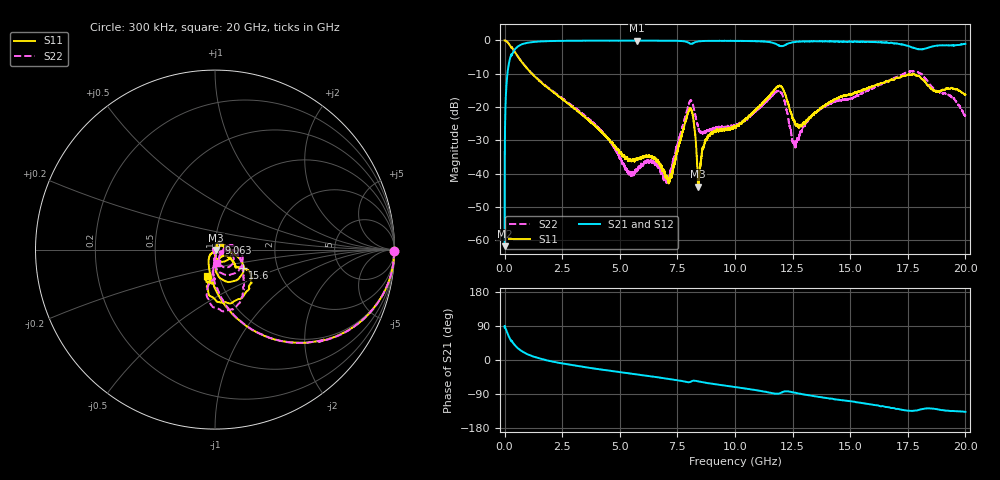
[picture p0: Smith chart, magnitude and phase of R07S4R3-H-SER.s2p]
!{R07S4R3}
!Johanson Technology Inc.
!www.johansontechnology.com
!Test Board Conditions:
!Substrate Type  RO4350B
!Substrate Thickness  10 mil
!Substrate Dk  3.66
!TL Type: GCPW
!TL Trace Width  21 mil
!TL Gap  20 mil
!Electrode orientation  Horizontal
!DUT TOPOLOGY	SERIES
!Mounting Pad LxW  16x21 mil
! Created Sat Feb  6 11:33:24 2021
# hz S ma R 50
! 2 Port Network Data from SP1.SP block
! freq  magS11  angS11  magS21  angS21  magS12  angS12  magS22  angS22
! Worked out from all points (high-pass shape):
!   20001 points, 300 kHz to 20 GHz, reference 50 ohm
!   highest |S21| = -0.04 dB at 5.74 GHz (marker M1); lowest = -61.7 dB at 300 kHz (marker M2)
!   |S21| within 3 dB of the highest: 408.8 MHz to end of sweep
!   lowest |S11| = -43.8 dB at 8.403 GHz (marker M3), VSWR 1.01, Z = 50.6 - j0.231 ohm
!   |S11| at or under -10 dB: 1.19 GHz to end of sweep
!   |S22| runs from -42.8 to 0.0 dB; largest |S21 - S12| = 0.013
!   S11 on the Smith chart (normalised r, x): 300 kHz: open; 9.063 GHz: 1.04, +0.08; 15.6 GHz: 1.33, -0.28; 20 GHz: 0.88, -0.26
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300000  0.9998 -0.5  0.0008196 86.0  0.00085 84.6  1 -0.6
1.163e8  0.9523 -18.5  0.3014 71.8  0.3017 71.7  0.9524 -18.4
3.463e8  0.7574 -42.6  0.6424 46.9  0.6437 47.0  0.7574 -42.5
1.1543e9  0.3255 -78.9  0.9402 11.2  0.9403 11.1  0.3293 -77.8
3.3343e9  0.0784 -116.8  0.9916 -17.4  0.9917 -17.4  0.08231 -94.5
5.4083e9  0.01628 -103.7  0.9934 -35.4  0.9939 -35.4  0.01018 -147.0
5.7403e9  0.0164 -81.2  0.9953 -38.1  0.9939 -38.1  0.01115 171.0
6.6673e9  0.01551 -64.4  0.9928 -45.8  0.9926 -45.9  0.01226 132.8
7.1843e9  0.008988 2.2  0.9909 -50.3  0.9897 -50.3  0.01005 39.3
8.0543e9  0.0953 -22.9  0.8957 -58.0  0.8962 -58.0  0.1249 -35.2
8.2063e9  0.06073 -72.9  0.918 -54.5  0.9178 -54.6  0.09903 -68.1
8.4033e9  0.006436 -20.8  0.9673 -56.3  0.9661 -56.4  0.04869 -62.9
8.6733e9  0.02803 65.2  0.9819 -59.5  0.9817 -59.5  0.04272 -39.2
9.0633e9  0.04231 60.8  0.9864 -63.3  0.9858 -63.3  0.04845 -26.0
1.00003e10  0.05022 23.0  0.9871 -71.3  0.9859 -71.4  0.05113 2.3
1.19033e10  0.2057 -47.4  0.8395 -88.5  0.8411 -88.5  0.1764 -42.0
1.25683e10  0.06134 -76.4  0.9429 -86.0  0.9461 -86.0  0.02871 -54.8
1.33343e10  0.07451 -29.0  0.9709 -94.3  0.9709 -94.4  0.07483 -2.8
1.56043e10  0.1844 -33.7  0.954 -114.5  0.9557 -114.5  0.1654 -26.7
1.66673e10  0.243 -35.5  0.9144 -124.7  0.9183 -125.1  0.2506 -50.1
1.79153e10  0.2972 -84.1  0.7435 -132.9  0.7479 -133.0  0.3396 -84.6
2e10  0.1524 -107.7  0.8918 -136.8  0.8881 -136.7  0.07512 -81.8
